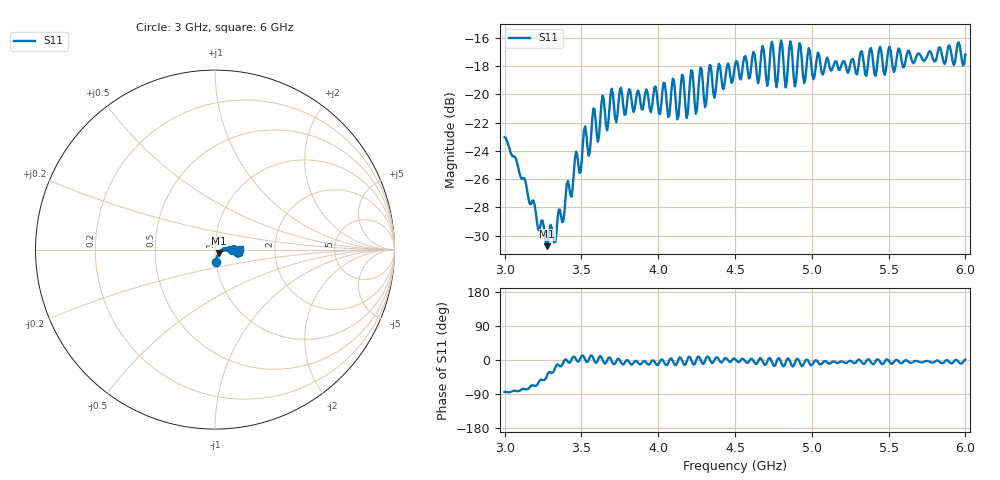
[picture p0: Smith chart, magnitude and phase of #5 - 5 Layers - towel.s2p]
!  02/07/2025  17:34:00
! Ref Plane: 0.000 mm
# MHZ S MA R  50
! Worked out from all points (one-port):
!   401 points, 3 GHz to 6 GHz, reference 50 ohm
!   lowest |S11| = -30.7 dB at 3.277 GHz (marker M1), VSWR 1.06, Z = 52.2 - j1.93 ohm
!   |S11| at or under -10 dB: start of sweep to end of sweep
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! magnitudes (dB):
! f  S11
! 3 GHz  -23.0
! 3.277 GHz  -30.7
! 3.375 GHz  -29.0
! 3.578 GHz  -21.0
! 3.607 GHz  -23.3
! 3.638 GHz  -20.1
! 3.667 GHz  -22.5
! 3.697 GHz  -19.6
! 3.728 GHz  -22.0
! 3.75 GHz  -19.7
! 4.005 GHz  -21.4
! 4.035 GHz  -19.2
! 4.065 GHz  -21.6
! 4.095 GHz  -18.9
! 4.125 GHz  -21.8
! 4.155 GHz  -18.6
! 4.185 GHz  -21.7
! 4.215 GHz  -18.3
! 4.245 GHz  -21.4
! 4.275 GHz  -18.1
! 4.305 GHz  -20.9
! 4.335 GHz  -17.9
! 4.365 GHz  -20.2
! 4.5 GHz  -17.9
! 4.875 GHz  -17.6
! 5.25 GHz  -17.9
! 5.625 GHz  -16.9
! 6 GHz  -17.2
